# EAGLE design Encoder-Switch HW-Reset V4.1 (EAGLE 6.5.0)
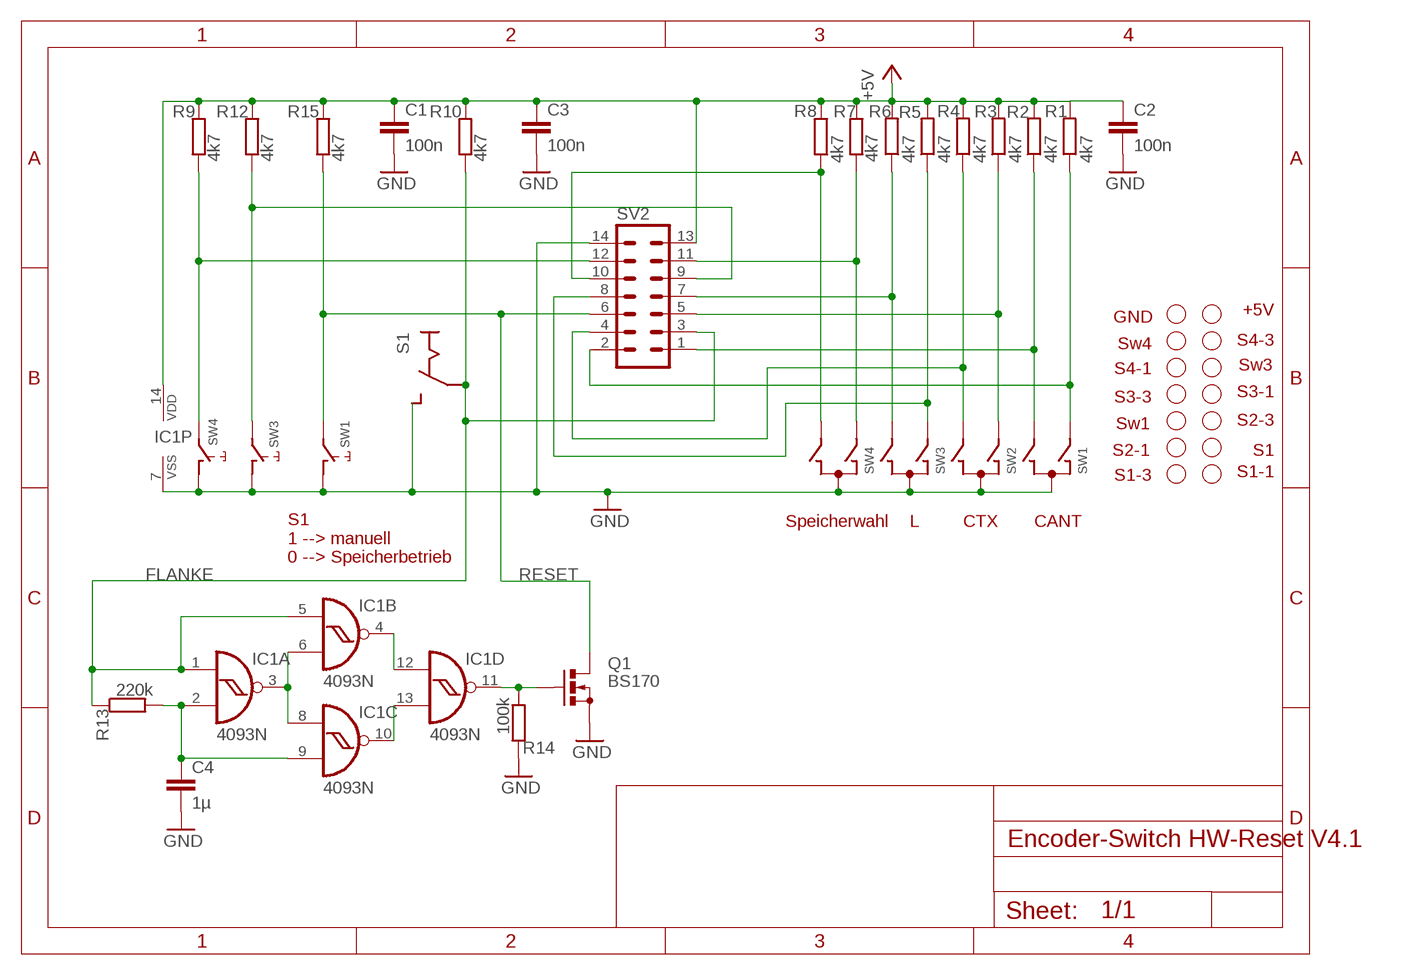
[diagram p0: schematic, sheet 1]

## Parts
C1  100n  C-EU025-025X050  [C025-025X050]
C2  100n  C-EU025-025X050  [C025-025X050]
C3  100n  C-EU025-025X050  [C025-025X050]
C4  1µ  C-EU050-045X075  [C050-045X075]
IC1  4093N  [DIL14]
Q1  BS170  [SOT54E]
R1  4k7  R-EU_0207/7  [0207/7]
R2  4k7  R-EU_0207/7  [0207/7]
R3  4k7  R-EU_0207/7  [0207/7]
R4  4k7  R-EU_0207/7  [0207/7]
R5  4k7  R-EU_0207/7  [0207/7]
R6  4k7  R-EU_0207/7  [0207/7]
R7  4k7  R-EU_0207/7  [0207/7]
R8  4k7  R-EU_0207/7  [0207/7]
R9  4k7  R-EU_0207/7  [0207/7]
R10  4k7  R-EU_0207/7  [0207/7]
R12  4k7  R-EU_0207/7  [0207/7]
R13  220k  R-EU_0207/7  [0207/7]
R14  100k  R-EU_0207/7  [0207/7]
R15  4k7  R-EU_0207/7  [0207/7]
S1  EIN-RAST  [EIN-RAST]
SV2  MA07-2  [MA07-2]
SW1  EC12E_SW  [ALPS_EC12E_SW]
SW2  EC12E_SW  [ALPS_EC12E_SW]
SW3  EC12E_SW  [ALPS_EC12E_SW]
SW4  EC12E_SW  [ALPS_EC12E_SW]

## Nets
+5V: C1.1 C2.1 C3.1 IC1.14(P:VDD) R1.2 R2.2 R3.2 R4.2 R5.2 R6.2 R7.1 R8.1 R9.1 R10.1 R12.1 R15.1 SV2.13
FLANKE: IC1.1(A:I0) IC1.5(B:I0) R10.2 R13.1 S1.M SV2.3
GND: C1.2 C2.2 C3.2 C4.2 IC1.7(P:VSS) Q1.S R14.1 S1.S SV2.14 SW1.C SW1.D SW2.C SW3.C SW3.D SW4.C SW4.D
N$1: R1.1 SV2.2 SW1.A
N$2: R7.2 SV2.11 SW4.A
N$3: R8.2 SV2.10 SW4.B
N$4: R9.2 SV2.12 SW4.E
N$5: R2.1 SV2.1 SW1.B
N$6: IC1.11(D:O) Q1.G R14.2
N$7: R12.2 SV2.9 SW3.E
N$10: R5.1 SV2.8 SW3.A
N$11: R3.1 SV2.5 SW2.A
N$12: R4.1 SV2.4 SW2.B
N$13: R6.1 SV2.7 SW3.B
N$15: C4.1 IC1.2(A:I1) IC1.9(C:I1) R13.2
N$18: IC1.3(A:O) IC1.6(B:I1) IC1.8(C:I0)
N$19: IC1.10(C:O) IC1.13(D:I1)
N$20: IC1.4(B:O) IC1.12(D:I0)
RESET: Q1.D R15.2 SV2.6 SW1.E
Unconnected: SW1.GND1(G) SW1.GND2(G) SW2.D SW2.E SW2.GND1(G) SW2.GND2(G) SW3.GND1(G) SW3.GND2(G) SW4.GND1(G) SW4.GND2(G)

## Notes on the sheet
- +5V
- GND
- Sw4 | S4-3
- S4-1 | Sw3
- S3-1
- S3-3
- Sw1 | S2-3
- S2-1 | S1
- S1-3 | S1-1
- Speicherwahl | L | CTX | CANT
- S1
  1 --> manuell
  0 --> Speicherbetrieb

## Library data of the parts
C1-C4 = rcl:C-EU: CAPACITOR, European symbol
IC1 = 40xx:4093: Quad 2-input NAND schmitt trigger
Q1 = transistor-small-signal:BS170: N-CHANNEL MOS FET
R1-R10 R12-R15 = rcl:R-EU_: RESISTOR, European symbol
S1 = eigen_2:EIN-RAST
SV2 = con-lstb:MA07-2: PIN HEADER
SW1-SW4 = switch-alps:EC12E_SW: ALPS rotary Encoder EC12E series with switch

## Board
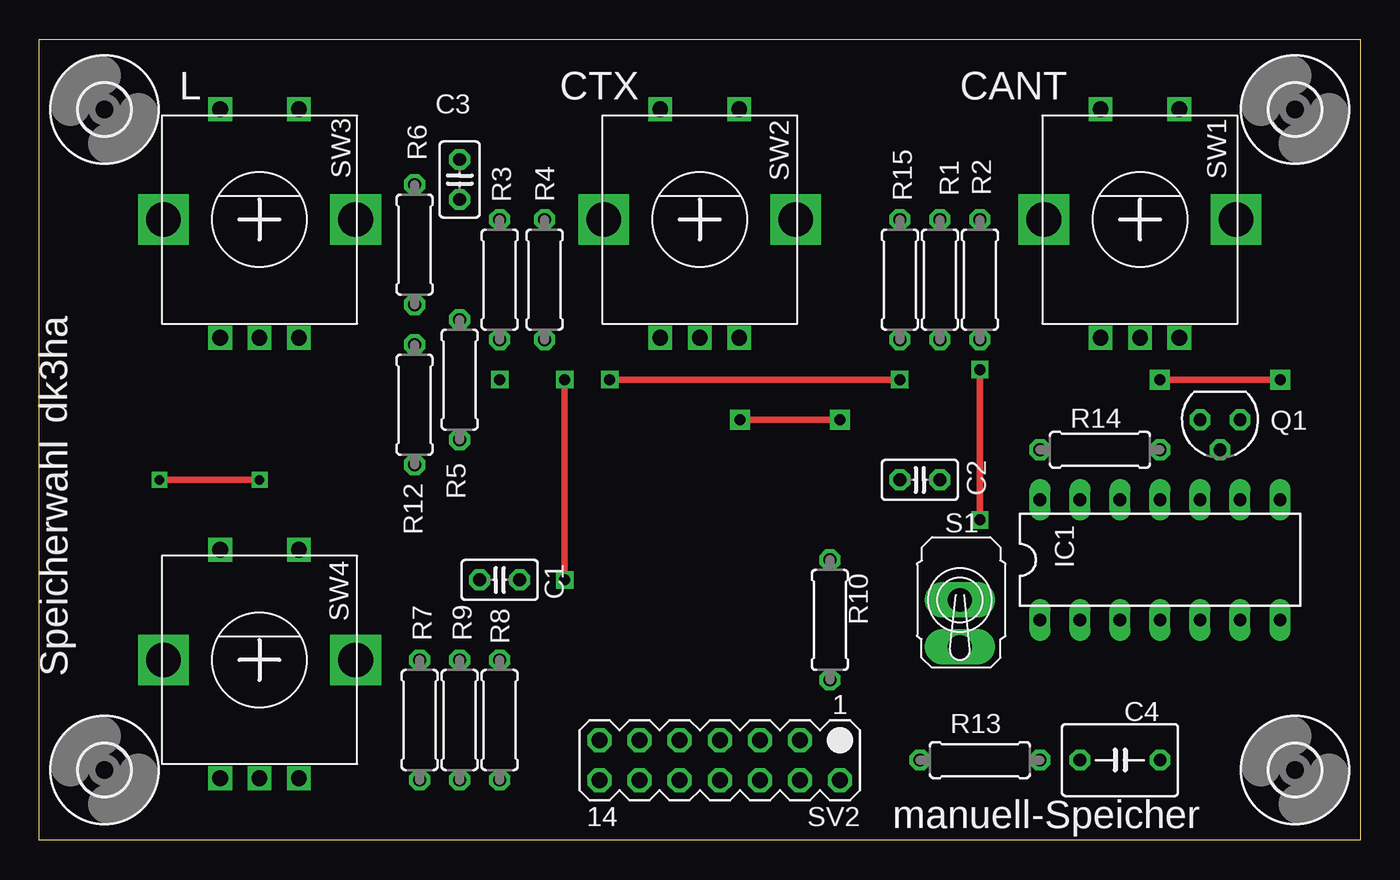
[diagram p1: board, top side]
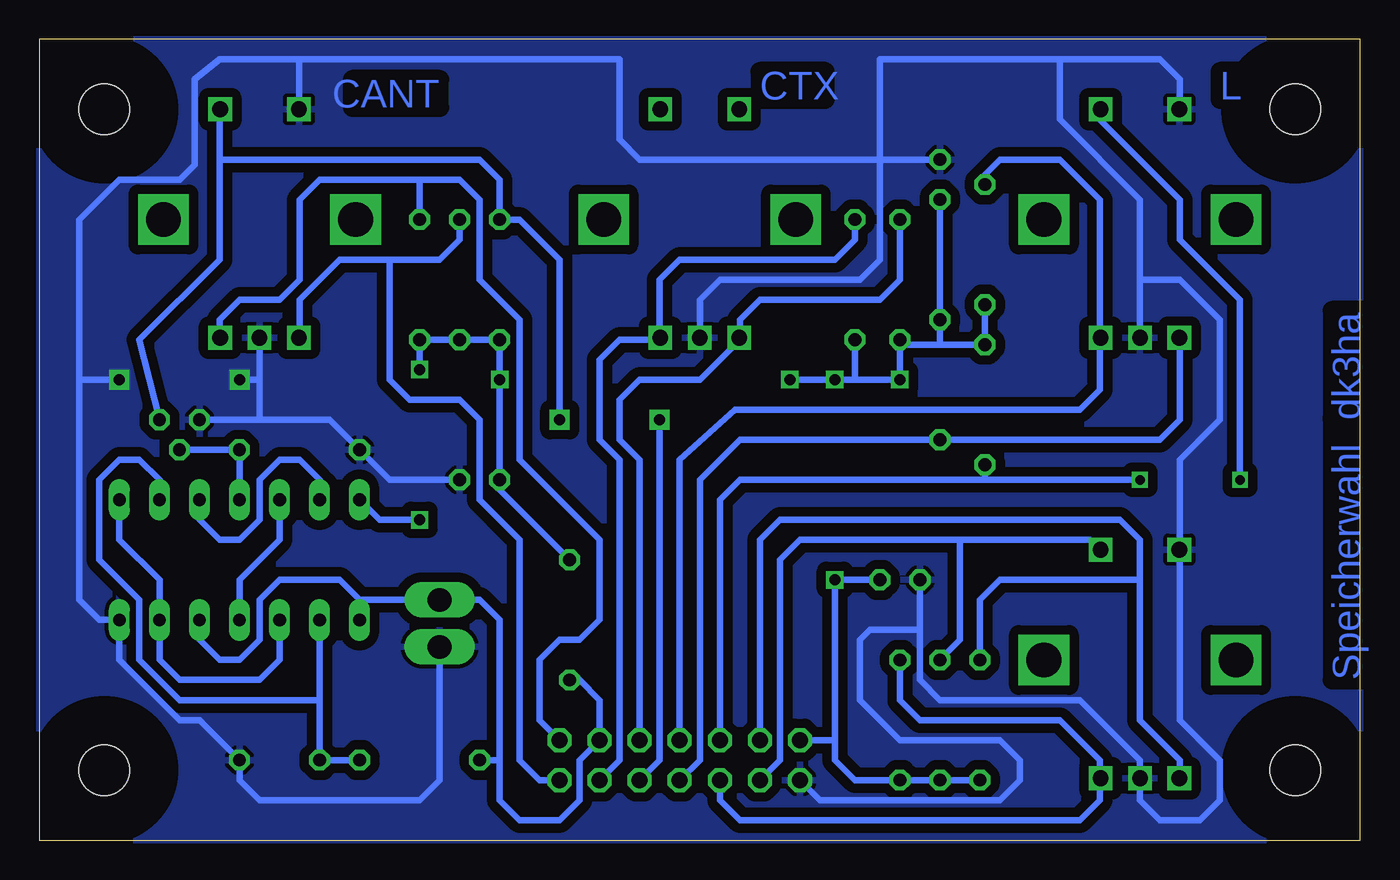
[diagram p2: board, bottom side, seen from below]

Size 83.82 x 50.8 mm. Coordinates in mm from the lower left corner, seen from the top.
Outline: 83.82,50.8 83.82,0 0,0 0,50.8 83.82,50.8
Copper layers (1*16): Top 0.035mm / dielectric 1.5mm / Bottom 0.035mm
Design rules "default *": minimum track width 16mil, minimum drill 24mil, track to track 8mil, track to pad 8mil, pad to pad 8mil, via to via 8mil, smd to smd 8mil, copper to edge 0mil, drill to drill 8mil, minimum pad ring 10mil, minimum via ring 8mil, stop-mask expansion 4mil, vias tented up to drill 0mil, thermal gap 10mil

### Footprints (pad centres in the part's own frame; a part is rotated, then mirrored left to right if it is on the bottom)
C025-025X050 = drill 0.813 octagon: 1 -1.27,0; 2 1.27,0
C050-045X075 = drill 0.813 octagon: 1 -2.54,0; 2 2.54,0
DIL14 = drill 0.813 long: 1 -7.62,-3.81; 2 -5.08,-3.81; 3 -2.54,-3.81; 4 0,-3.81; 5 2.54,-3.81; 6 5.08,-3.81; 7 7.62,-3.81; 8 7.62,3.81; 9 5.08,3.81; 10 2.54,3.81; 11 0,3.81; 12 -2.54,3.81; 13 -5.08,3.81; 14 -7.62,3.81
SOT54E = drill 0.813 octagon: D -1.27,0; G 0,1.905; S 1.27,0
0207/7 = drill 0.813 octagon: 1 -3.81,0; 2 3.81,0
EIN-RAST = drill 1.5 pad 2.184 long: M 0,0; S 0,-2.982
MA07-2 = drill 1.016 octagon: 1 -7.62,-1.27; 2 -7.62,1.27; 3 -5.08,-1.27; 4 -5.08,1.27; 5 -2.54,-1.27; 6 -2.54,1.27; 7 0,-1.27; 8 0,1.27; 9 2.54,-1.27; 10 2.54,1.27; 11 5.08,-1.27; 12 5.08,1.27; 13 7.62,-1.27; 14 7.62,1.27
ALPS_EC12E_SW = drill 1 square: A -2.5,-7.5; B 2.5,-7.5; C 0,-7.5; D -2.5,7; E 2.5,7 | drill 2.2 square: GND1 -6.1,0; GND2 6.1,0
3,2 = hole 3.2: 0,0

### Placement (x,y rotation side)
C1  29.21,16.51 180 top
C2  55.88,22.86 0 top
C3  26.67,41.91 90 top
C4  68.58,5.08 0 top
IC1  71.12,17.78 0 top
Q1  74.93,26.67 180 top
R1  57.15,35.56 270 top
R2  59.69,35.56 270 top
R3  29.21,35.56 270 top
R4  32.07,35.56 270 top
R5  26.67,29.21 90 top
R6  23.81,37.78 270 top
R7  24.13,7.62 90 top
R8  29.21,7.62 90 top
R9  26.67,7.62 90 top
R10  50.16,13.97 270 top
R12  23.81,27.62 270 top
R13  59.69,5.08 0 top
R14  67.31,24.77 0 top
R15  54.61,35.56 90 top
S1  58.42,15.24 0 top
SV2  43.18,5.08 180 top
SW1  69.85,39.37 0 top
SW2  41.91,39.37 0 top
SW3  13.97,39.37 0 top
SW4  13.97,11.43 0 top
U$1  [3,2]  4.13,4.45 270 top
U$5  [3,2]  4.13,46.35 270 top
U$6  [3,2]  79.69,4.45 270 top
U$7  [3,2]  79.69,46.35 270 top

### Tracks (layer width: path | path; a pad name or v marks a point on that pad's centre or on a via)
+5V  (via drill 0.7, 0.7 pad 1.02)
  Top 0.406: v36.2,29.21 v54.61,29.21 | v33.34,16.51 v33.34,29.21 | v59.69,20.32 v59.69,29.84
  Bottom 0.406: R7.1 R9.1 R8.1 32.07,3.81 33.34,5.08 33.34,6.35 | 32.07,29.21 v29.21,29.21 R3.2 28.89,31.43 26.67,31.43 | 32.07,29.21 v33.34,29.21 v36.2,29.21 | SV2.13 33.34,6.35 | 33.34,6.35 v33.34,16.51 C1.1 | IC1.14 62.23,20.32 v59.69,20.32 | v59.69,29.84 R2.2 R1.2 R15.1 v54.61,29.21 C2.1 54.61,22.23 R10.1 | R4.2 32.07,29.21 | 26.67,31.43 R12.1 R6.2 | 26.67,31.43 R5.2 C3.1
FLANKE
  Bottom 0.406: R10.2 49.53,10.16 48.26,8.89 SV2.3 49.53,5.08 49.53,2.54 50.8,1.27 53.34,1.27 54.61,2.54 54.61,5.08 | 54.61,5.08 54.61,13.97 55.88,15.24 S1.M 63.5,15.24 | IC1.5 73.66,12.7 72.39,11.43 71.12,11.43 69.85,12.7 69.85,15.24 68.58,16.51 64.77,16.51 63.5,15.24 | 63.5,15.24 IC1.1 | R13.1 54.61,5.08
GND  (via drill 0.7 pad 1.27)
  Top 0.406: v78.74,29.21 v71.12,29.21
  Bottom 0.406: 19.05,49.53 12.7,49.53 11.43,48.26 11.43,46.35 11.41,46.37 SW3.D | 19.05,49.53 30.48,49.53 30.48,43.18 | SW2.C 41.91,34.29 40.64,35.56 31.75,35.56 30.48,36.83 30.48,43.18 | C3.2 30.48,43.18 | SV2.14 34.29,2.54 22.86,2.54 21.59,3.81 21.59,5.08 22.86,6.35 29.21,6.35 31.75,8.89 31.75,12.7 31.11,13.34 27.94,13.34 | 27.94,13.34 27.94,10.16 26.67,8.89 17.78,8.89 13.97,5.08 SW4.C 13.97,2.54 12.7,1.27 10.16,1.27 8.89,2.54 8.89,5.08 11.43,7.62 11.43,18.39 SW4.D 11.43,18.47 11.43,24.13 8.89,26.67 8.89,33.02 11.43,35.56 13.97,35.56 | S1.S 58.42,3.81 59.69,2.54 69.85,2.54 71.12,3.81 C4.2 73.66,7.62 74.93,7.62 78.74,11.43 IC1.7 80.01,13.97 81.28,15.24 81.28,29.21 | C2.2 61.59,22.86 R14.1 65.41,26.67 69.85,26.67 | 67.31,49.53 46.99,49.53 46.99,44.45 45.72,43.18 30.48,43.18 | 67.31,49.53 72.39,49.53 73.98,48.26 73.98,42.86 74.93,41.91 78.74,41.91 81.28,39.37 81.28,29.21 | C1.2 27.94,13.34 | SW1.D 67.35,49.49 67.31,49.53 | Q1.S 69.85,26.67 | 81.28,29.21 v78.74,29.21 | SW1.C 69.85,29.21 | 69.85,29.21 69.85,26.67 | v71.12,29.21 69.85,29.21 | SW3.C 13.97,35.56 | 13.97,35.56 13.97,40.64 19.05,45.72 19.05,49.53
  pour Bottom (isolate 0.61): 83.82,50.8 83.82,0 0,0 0,50.8
N$1
  Bottom 0.406: SV2.2 52.07,3.81 53.34,5.08 53.34,19.05 55.88,21.59 55.88,26.67 57.15,27.94 60.33,27.94 61.59,29.21 61.59,36.83 | SW1.A 67.31,31.83 67.31,34.29 64.77,36.83 61.59,36.83 | R1.1 57.15,38.1 58.42,36.83 61.59,36.83
N$2
  Bottom 0.406: 13.97,16.51 13.97,7.62 11.43,5.08 11.43,3.97 SW4.A | SV2.11 38.1,19.05 36.83,20.32 15.24,20.32 13.97,19.05 13.97,16.51 | R7.2 24.13,15.24 22.86,16.51 13.97,16.51
N$3
  Bottom 0.406: R8.2 29.21,8.89 27.94,7.62 19.05,7.62 16.51,5.08 16.51,3.97 SW4.B 16.51,3.89 16.51,2.54 17.78,1.27 39.37,1.27 40.64,2.54 SV2.10
N$4
  Bottom 0.406: R9.2 25.4,12.7 25.4,19.05 | 25.4,19.05 17.14,19.05 16.51,18.41 16.51,18.39 SW4.E | SV2.12 36.83,5.08 36.83,17.78 35.56,19.05 25.4,19.05
N$5
  Bottom 0.406: 72.39,31.75 72.39,31.83 | 72.39,31.83 SW1.B 72.39,31.91 | 72.39,31.83 72.39,31.91 | SV2.1 52.07,7.62 52.07,11.43 50.8,12.7 49.53,12.7 48.26,13.97 48.26,19.05 53.34,24.13 53.34,33.02 55.88,35.56 55.88,40.64 57.15,41.91 59.69,41.91 | 59.69,41.91 66.04,41.91 67.31,40.64 67.31,35.56 68.58,34.29 71.12,34.29 72.39,33.02 72.39,31.91 | R2.1 59.69,41.91
N$6
  Bottom 0.406: Q1.G R14.2 IC1.11
N$7  (via drill 0.6)
  Top 0.406: v7.62,22.86 v13.97,22.86
  Bottom 0.406: SV2.9 40.64,21.59 39.37,22.86 23.81,22.86 | SW3.E 16.47,45.68 11.43,40.64 11.43,38.1 7.62,34.29 v7.62,22.86 | v13.97,22.86 23.81,22.86 | 23.81,22.86 R12.2
N$10
  Bottom 0.406: 11.43,31.91 SW3.A 11.43,31.83 11.43,26.67 12.7,25.4 R5.1 39.37,25.4 41.91,22.86 41.91,5.08 SV2.8
N$11
  Bottom 0.406: R3.1 29.21,35.56 30.48,34.29 38.1,34.29 39.37,33.02 39.37,31.91 SW2.A 39.37,31.83 39.37,31.75 41.91,29.21 45.72,29.21 46.99,27.94 46.99,25.4 45.72,24.13 SV2.5
N$12
  Bottom 0.406: R4.1 32.07,38.1 33.34,36.83 43.18,36.83 44.45,35.56 44.45,31.91 SW2.B 44.53,31.75 46.99,31.75 48.26,30.48 48.26,25.4 46.99,24.13 46.99,5.08 SV2.4
N$13
  Bottom 0.406: SV2.7 43.18,24.13 39.69,27.3 17.78,27.3 16.51,28.57 16.51,31.83 SW3.B 16.51,31.91 16.51,40.64 19.05,43.18 22.86,43.18 23.81,42.23 R6.1
N$15
  Bottom 0.406: IC1.9 76.2,22.86 77.47,24.13 78.74,24.13 80.01,22.86 80.01,17.78 77.47,15.24 77.47,11.43 74.93,8.89 66.04,8.89 | 66.04,8.89 C4.1 R13.2 | 66.04,8.89 IC1.2
N$18
  Bottom 0.406: IC1.8 78.74,19.05 76.2,16.51 IC1.6 76.2,11.43 74.93,10.16 69.85,10.16 68.58,11.43 IC1.3
N$19
  Bottom 0.406: IC1.13 66.04,22.86 67.31,24.13 68.58,24.13 69.85,22.86 69.85,20.32 71.12,19.05 72.39,19.05 73.66,20.32 IC1.10
N$20
  Bottom 0.406: IC1.4 71.12,16.51 68.58,19.05 IC1.12
RESET  (via drill 0.7 pad 1.27)
  Top 0.406: v50.8,26.67 v44.45,26.67
  Bottom 0.406: SV2.6 44.45,5.08 v44.45,26.67 | 72.39,43.18 55.88,43.18 54.61,41.91 R15.2 53.34,39.37 50.8,36.83 v50.8,26.67 | 72.39,43.18 72.39,46.33 SW1.E | Q1.D 77.47,31.75 72.39,36.83 72.39,43.18

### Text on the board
Bottom: CANT | L | CTX | dk3ha | Speicherwahl
tPlace: L | CTX | CANT | dk3ha | Speicherwahl | manuell-Speicher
